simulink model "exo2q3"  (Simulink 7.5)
settings: Solver=ode45  StartTime=0.0  StopTime=20  RelTol=1e-3
libraries: fuzblock x2, simulink x1

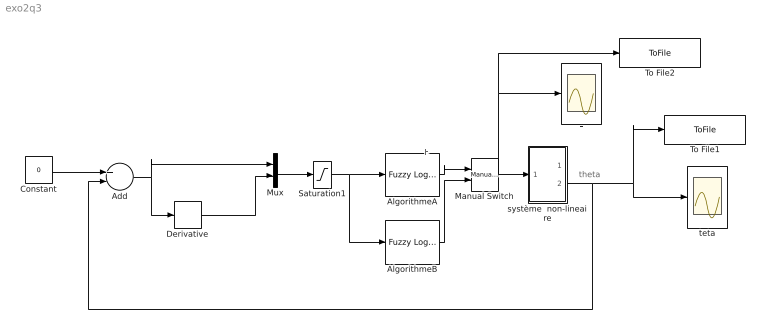
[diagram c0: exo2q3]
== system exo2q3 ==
  note: theta
  note: F
  Add : Sum  Inputs=+-  OutDataType=fixdt(1, 16)  OutScaling=2^-10
  AlgorithmeA : fuzblock/Fuzzy Logic  Controller  SystemSampleTime=-1  fis=flouA
  AlgorithmeB : fuzblock/Fuzzy Logic  Controller  SystemSampleTime=-1  fis=flouB
  Constant : Constant  Value=0  OutDataType=fixdt(1, 16)  OutScaling=2^0
  Derivative : Derivative
  F : Scope
  Manual Switch : simulink/Signal Routing/Manual Switch  SystemSampleTime=-1  sw=0  action=0  varsize=off
  Mux : Mux  Inputs=2
  Saturation1 : Saturate  UpperLimit=0.3  LowerLimit=-0.3  OutDataType=fixdt(1, 16)  OutScaling=2^0
  To File1 : ToFile  Filename=pendulespace
  To File2 : ToFile  Filename=flou
  système  non-lineaire : Subsystem
  teta : Scope
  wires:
  Constant/1 -> Add/1
  Add/1 -> Derivative/1, Mux/1
  Derivative/1 -> Mux/2
  système  non-lineaire/2(Out2) -> Add/2, teta/1, To File1/1
  Mux/1 -> Saturation1/1
  Manual Switch/1 -> système  non-lineaire/1(In1), F/1, To File2/1
  AlgorithmeA/1 -> Manual Switch/1
  AlgorithmeB/1 -> Manual Switch/2
  Saturation1/1 -> AlgorithmeA/1, AlgorithmeB/1

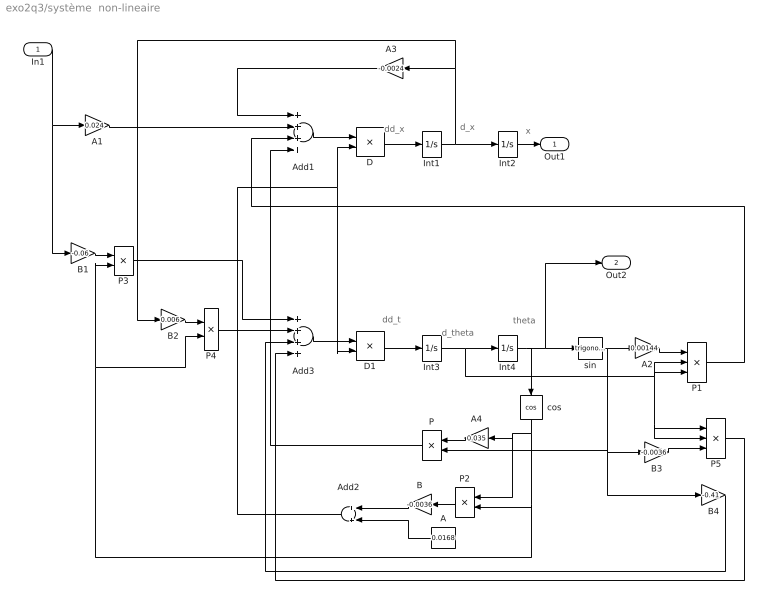
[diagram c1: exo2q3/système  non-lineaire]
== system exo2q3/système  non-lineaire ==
  note: d_x
  note: x
  note: theta
  note: d_theta
  note: dd_t
  note: dd_x
  In1 : Inport  OutDataType=fixdt(1, 16)  OutScaling=2^0
  A : Constant  Value=0.0168  OutDataType=fixdt(1, 16)  OutScaling=2^0
  A1 : Gain  Gain=0.024  ParameterDataType=fixdt(1, 16)  ParameterScaling=2^0  OutDataType=fixdt(1, 16)  OutScaling=2^0
  A2 : Gain  Gain=0.00144  ParameterDataType=fixdt(1, 16)  ParameterScaling=2^0  OutDataType=fixdt(1, 16)  OutScaling=2^0
  A3 : Gain  Gain=-0.0024  ParameterDataType=fixdt(1, 16)  ParameterScaling=2^0  OutDataType=fixdt(1, 16)  OutScaling=2^0
  A4 : Gain  Gain=0.035  ParameterDataType=fixdt(1, 16)  ParameterScaling=2^0  OutDataType=fixdt(1, 16)  OutScaling=2^0
  Add1 : Sum  Inputs=++++  OutDataType=fixdt(1, 16)  OutScaling=2^-10
  Add2 : Sum  OutDataType=fixdt(1, 16)  OutScaling=2^-10
  Add3 : Sum  Inputs=++++  OutDataType=fixdt(1, 16)  OutScaling=2^-10
  B : Gain  Gain=-0.0036  ParameterDataType=fixdt(1, 16)  ParameterScaling=2^0  OutDataType=fixdt(1, 16)  OutScaling=2^0
  B1 : Gain  Gain=-0.06  ParameterDataType=fixdt(1, 16)  ParameterScaling=2^0  OutDataType=fixdt(1, 16)  OutScaling=2^0
  B2 : Gain  Gain=0.006  ParameterDataType=fixdt(1, 16)  ParameterScaling=2^0  OutDataType=fixdt(1, 16)  OutScaling=2^0
  B3 : Gain  Gain=-0.0036  ParameterDataType=fixdt(1, 16)  ParameterScaling=2^0  OutDataType=fixdt(1, 16)  OutScaling=2^0
  B4 : Gain  Gain=-0.41  ParameterDataType=fixdt(1, 16)  ParameterScaling=2^0  OutDataType=fixdt(1, 16)  OutScaling=2^0
  D : Product  Inputs=*/  OutDataType=fixdt(1, 16)  OutScaling=2^-10
  D1 : Product  Inputs=*/  OutDataType=fixdt(1, 16)  OutScaling=2^-10
  Int{1..4} (4 alike) : Integrator  InitialCondition=1
  P{,2..4} (4 alike) : Product  OutDataType=fixdt(1, 16)  OutScaling=2^0
  P1 : Product  Inputs=3  OutDataType=fixdt(1, 16)  OutScaling=2^0
  P5 : Product  Inputs=3  OutDataType=fixdt(1, 16)  OutScaling=2^0
  cos : Trigonometry  Operator=cos
  sin : Trigonometry
  Out1 : Outport
  Out2 : Outport  Port=2  OutDataType=fixdt(1, 16)  OutScaling=2^0
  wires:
  A1/1 -> Add1/2
  Int4/1 -> cos/1, sin/1, Out2/1
  sin/1 -> A2/1, P/2, B3/1, B4/1
  Int3/1 -> Int4/1, P1/3, P1/2, P5/2, P5/1
  A2/1 -> P1/1
  P1/1 -> Add1/3
  Int1/1 -> Int2/1, A3/1, B2/1
  A3/1 -> Add1/1
  cos/1 -> A4/1, P2/1, P2/2, P3/2, P4/2
  A4/1 -> P/1
  P/1 -> Add1/4
  P2/1 -> B/1
  B/1 -> Add2/1
  A/1 -> Add2/2
  Add1/1 -> D/1
  Add2/1 -> D/2, D1/2
  D/1 -> Int1/1
  B1/1 -> P3/1
  B2/1 -> P4/1
  B3/1 -> P5/3
  P3/1 -> Add3/1
  P4/1 -> Add3/2
  B4/1 -> Add3/3
  P5/1 -> Add3/4
  Add3/1 -> D1/1
  D1/1 -> Int3/1
  In1/1 -> A1/1, B1/1
  Int2/1 -> Out1/1
